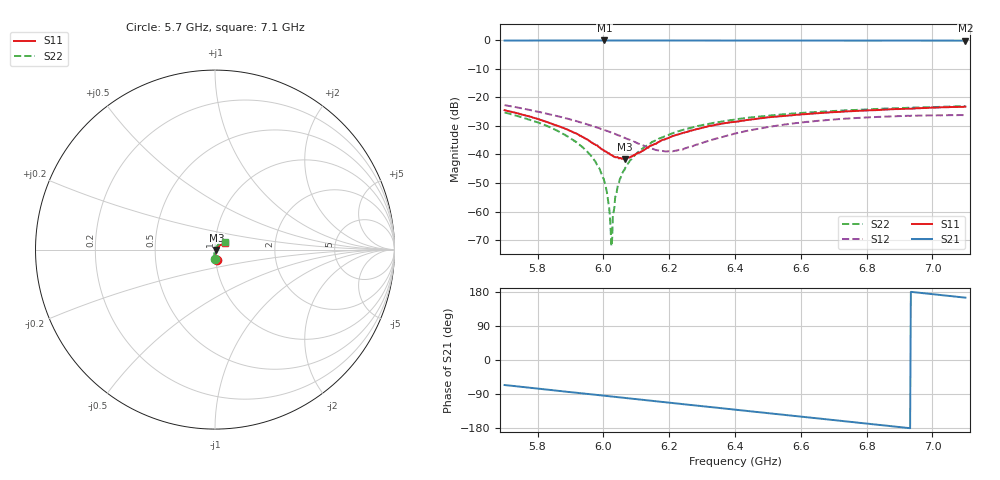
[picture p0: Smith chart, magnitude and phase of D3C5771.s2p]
! 4/14/2021 3:10:29 PM
! C:\USERS\DITOM\DESKTOP\SINGLE JUNCTION ISOLATOR DATA\5.7-7.1 GHZ (D3I5771).S2P
! CHANNEL.1
! TR.MEASUREMENT
! CORRECTED.DATA
# GHZ S RI R 50.0
! FREQ.GHZ  S11RE  S11IM  S21RE  S21IM  S12RE  S12IM  S22RE  S22IM
!; PortSelection: Port_12
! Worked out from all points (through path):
!   601 points, 5.7 GHz to 7.1 GHz, reference 50 ohm
!   highest |S21| = -0.07 dB at 6.003 GHz (marker M1); lowest = -0.1 dB at 7.1 GHz (marker M2)
!   lowest |S11| = -41.5 dB at 6.066 GHz (marker M3), VSWR 1.02, Z = 50.8 - j0.215 ohm
!   |S11| at or under -10 dB: start of sweep to end of sweep
!   |S22| runs from -72.1 to -23.1 dB; largest |S21 - S12| = 1.1
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5.7  0.0109 -0.0587  0.4005 -0.9029  -0.0553 0.0477  0.00127 -0.0545
5.830667  0.00472 -0.0363  0.2021 -0.97  -0.0244 0.0453  -0.0041 -0.0308
5.889  0.00389 -0.0273  0.1065 -0.9848  -0.0132 0.0404  -0.00432 -0.0206
5.935667  0.00451 -0.0198  0.0337 -0.9888  -0.00535 0.0353  -0.00357 -0.0131
5.973  0.00512 -0.0143  -0.0262 -0.9915  -0.00025 0.0306  -0.00248 -0.00745
5.994  0.00535 -0.0112  -0.0613 -0.99  0.00213 0.0278  -0.00173 -0.00432
6.003333  0.00573 -0.00992  -0.0766 -0.9894  0.00326 0.0266  -0.00131 -0.00307
6.012667  0.00616 -0.00874  -0.0921 -0.9874  0.00407 0.0253  -0.000825 -0.00169
6.019667  0.00622 -0.00799  -0.1032 -0.9862  0.00483 0.0243  -0.000489 -0.000704
6.026667  0.00647 -0.00714  -0.1144 -0.9846  0.00544 0.0232  -0.000257 0.0002
6.031333  0.00664 -0.00636  -0.1217 -0.9834  0.00605 0.0226  -2.02e-05 0.000995
6.036  0.00681 -0.00579  -0.129 -0.9822  0.00629 0.0219  0.000249 0.00178
6.043  0.00733 -0.00519  -0.1399 -0.9801  0.00677 0.0208  0.000588 0.0026
6.052333  0.00782 -0.00376  -0.1541 -0.9779  0.0075 0.0196  0.00112 0.00373
6.066333  0.0081 -0.00212  -0.176 -0.9743  0.00849 0.0174  0.00177 0.00549
6.103667  0.0103 0.00231  -0.2343 -0.9629  0.0102 0.0119  0.00383 0.0101
6.166667  0.0137 0.00889  -0.331 -0.9335  0.0115 0.00252  0.0081 0.0166
6.234333  0.018 0.0144  -0.431 -0.8918  0.0101 -0.00666  0.0132 0.0225
6.4  0.0282 0.0245  -0.6497 -0.7455  -0.00236 -0.0231  0.0254 0.032
6.635667  0.0414 0.0315  -0.877 -0.4539  -0.0298 -0.0235  0.0395 0.038
6.866667  0.0505 0.0351  -0.9813 -0.1051  -0.0463 0.000551  0.0489 0.0405
7.1  0.0575 0.0376  -0.9487 0.2626  -0.0358 0.0332  0.0561 0.0423
